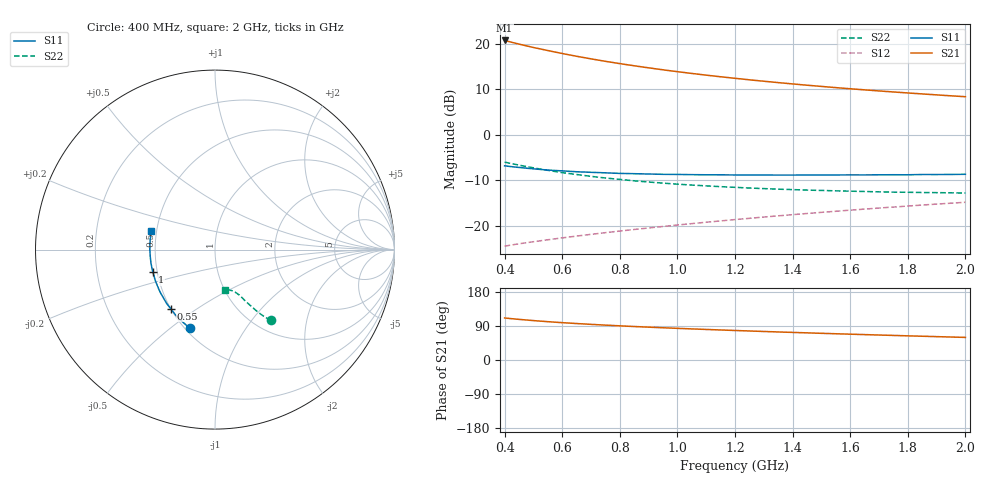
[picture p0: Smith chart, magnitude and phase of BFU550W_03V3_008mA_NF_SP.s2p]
! Filename:  P:\Prog\Test\Noise\ATS_data\Testdata_Net\06 Compressed Noise after Statistics\BFU550W_APM2013_11_D05_03p3V_008mA_NF_CM01_D.sf
! Date/Time: Tue 26/Mar/2013 16:25:27
! BFU550W_APM2013_11_D05_03p3V_1to35mA_NF_CM01_Bias5_R.sf
! Noise Parameter Data File
! BFU550W_APM2013_11_D05_03p3V_1to35mA_NF_CM01
! Date/time: Mon Mar 25 12:16:07 2013
! VAR V_out= 3.300000
! VAR I_out= 7.995000
! VAR V_in= 0.824300
! VAR I_in= 0.084600
! Device data file deembeded for feedlines and parallel
! Original file: \06 Compressed Noise after Statistics\BFU550W_APM2013_11_D05_03p3V_008mA_NF_CM01_R.sf
! Feed-files: PR019V01_070313_Feed1.s2p, PR019V01_070313_Feed2.s2p
! Parallel-file: PR019V01_070313_Par.s2p
# MHz S MA R 50
!  Freq-MHz  S11-mag  S11-arg  S21-mag  S21-arg  S12-mag  S12-arg  S22-mag  S22-arg
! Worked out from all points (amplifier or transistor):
!   37 points, 400 MHz to 2 GHz, reference 50 ohm
!   highest |S21| = 20.7 dB at 400 MHz (marker M1)
!   |S21| within 3 dB of that: start of sweep to 611.2 MHz
!   unconditionally stable (mu >= 1): 1.443 GHz to end of sweep
!   at 500 MHz: K = 0.68, MSG = 21.3 dB, |S12| = -23.4 dB
!   at 1.1 GHz: K = 0.95, MSG = 16.1 dB, |S12| = -19.2 dB
!   at 2 GHz: K = 1.02, MAG = 10.7 dB, |S12| = -14.8 dB
!   lowest NFmin = 0.65 dB at 433 MHz
!   S11 on the Smith chart (normalised r, x): 400 MHz: 0.53, -0.58; 550 MHz: 0.50, -0.40; 1 GHz: 0.47, -0.14; 2 GHz: 0.47, +0.11
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400  0.4578 -107.9  10.89 110.9  0.06009 55.7  0.5028 -51.7
420  0.45 -110.9  10.49 109.3  0.06162 55.6  0.4877 -52.5
433  0.4449 -112.7  10.24 108.4  0.06254 55.5  0.4782 -52.9
460  0.4365 -116.3  9.762 106.6  0.06448 55.5  0.4597 -53.8
500  0.4244 -121.4  9.12 104.0  0.06722 55.6  0.4353 -54.9
550  0.4112 -126.8  8.441 101.1  0.07064 55.9  0.4085 -56.1
600  0.4031 -132.1  7.834 98.5  0.07409 56.2  0.3855 -56.9
650  0.3942 -136.5  7.303 96.2  0.07755 56.6  0.3675 -57.8
700  0.3886 -140.8  6.841 94.0  0.08102 57.0  0.351 -58.5
750  0.3836 -144.6  6.431 92.0  0.08451 57.4  0.3367 -59.1
800  0.3782 -148.2  6.067 90.2  0.08808 57.8  0.3249 -59.9
850  0.3754 -151.7  5.743 88.3  0.09159 58.2  0.3135 -60.3
950  0.3694 -157.5  5.187 85.1  0.09888 59.0  0.2958 -61.4
1000  0.3685 -160.3  4.949 83.5  0.1025 59.3  0.288 -61.8
1100  0.3652 -165.3  4.533 80.6  0.11 59.9  0.2759 -63.0
1200  0.3636 -169.8  4.185 77.9  0.1177 60.3  0.2659 -64.3
1250  0.3629 -172.1  4.028 76.6  0.1215 60.4  0.2614 -64.7
1350  0.3624 -175.9  3.754 74.0  0.1294 60.7  0.2538 -66.0
1500  0.363 178.6  3.408 70.4  0.1413 60.9  0.2458 -68.2
1650  0.3639 173.5  3.124 67.0  0.1534 60.9  0.2393 -70.3
1750  0.3656 170.7  2.964 64.8  0.1615 60.8  0.2354 -72.0
2000  0.3698 163.5  2.629 59.6  0.1823 60.2  0.2303 -76.6
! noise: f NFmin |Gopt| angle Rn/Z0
400  0.6689  0.06565  124.7  0.0762
460  0.66  0.07886  132.6  0.0763
600  0.7124  0.08613  127.9  0.0799
800  0.7165  0.1387  141.9  0.0722
1000  0.7536  0.1728  149.4  0.067
1200  0.8159  0.2014  154.3  0.0651
1400  0.8211  0.2284  164.2  0.0651
1600  0.8543  0.2629  173.8  0.0569
1800  0.884  0.2952  180  0.0566
2000  0.9147  0.3094  -173.5  0.0601
